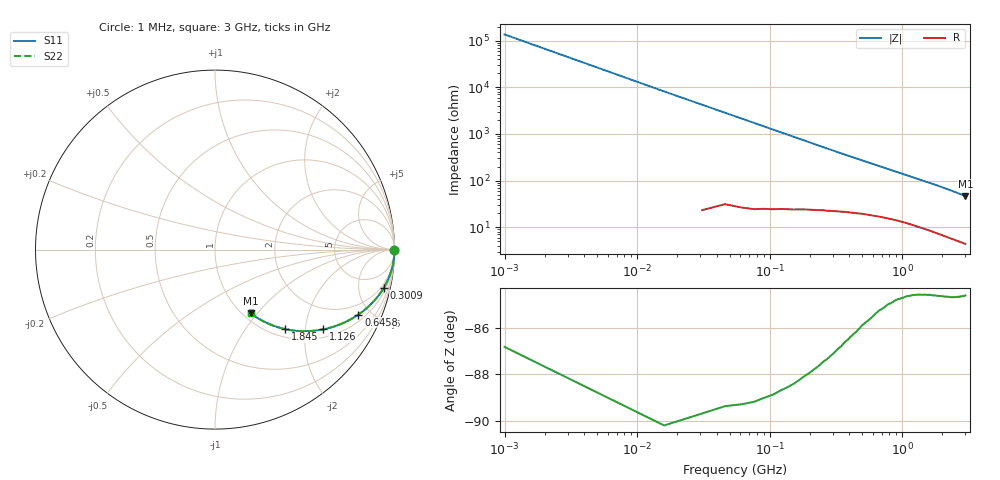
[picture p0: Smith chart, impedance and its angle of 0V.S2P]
!Keysight Technologies,E4991B,MY54301043,A.02.04
!Date: Thu Nov 16 21:16:10 2023
!Data:
!Freq	S11	S21	S12	S22
# Hz S MA R 50
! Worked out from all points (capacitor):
!   201 points, 1 MHz to 3 GHz, reference 50 ohm
!   read as one part in series: C = 1.22 pF near 15.99 MHz
!   lowest |Z| = 46.6 ohm at 3 GHz (marker M1)
!   S11 on the Smith chart (normalised r, x): 1 MHz: open; 300.9 MHz: 1.44, -8.79; 645.8 MHz: 1.35, -4.23; 1.126 GHz: 1.24, -2.51; 1.845 GHz: 1.15, -1.56; 3 GHz: 1.09, -0.93
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1000000  1 -0.0  0.0007395 86.8  0.0007395 86.8  1 -0.0
1.5995e7  1 -0.7  0.01229 89.5  0.01229 89.5  1 -0.7
3.099e7  0.9996 -1.4  0.02374 88.3  0.02374 88.3  0.9996 -1.4
4.5985e7  0.999 -2.0  0.03525 87.3  0.03525 87.3  0.999 -2.0
6.098e7  0.9983 -2.7  0.04665 86.6  0.04665 86.6  0.9983 -2.7
7.5975e7  0.9975 -3.3  0.0581 85.9  0.0581 85.9  0.9975 -3.3
1.05965e8  0.9951 -4.6  0.08074 84.2  0.08074 84.2  0.9951 -4.6
1.35955e8  0.9921 -5.9  0.1031 82.6  0.1031 82.6  0.9921 -5.9
1.65945e8  0.9883 -7.2  0.1251 81.1  0.1251 81.1  0.9883 -7.2
2.1093e8  0.9816 -9.1  0.1574 78.8  0.1574 78.8  0.9816 -9.1
3.009e8  0.9647 -12.6  0.2192 74.5  0.2192 74.5  0.9647 -12.6
3.9087e8  0.9443 -16.0  0.2764 70.5  0.2764 70.5  0.9443 -16.0
5.1083e8  0.9137 -20.1  0.3454 65.7  0.3454 65.7  0.9137 -20.1
6.45785e8  0.8772 -24.4  0.4137 61.0  0.4137 61.0  0.8772 -24.4
8.1073e8  0.8323 -28.9  0.4857 56.0  0.4857 56.0  0.8323 -28.9
1.005665e9  0.7805 -33.7  0.5571 51.0  0.5571 51.0  0.7805 -33.7
1.125625e9  0.7498 -36.3  0.5949 48.3  0.5949 48.3  0.7498 -36.3
1.5005e9  0.6615 -43.4  0.6897 41.2  0.6897 41.2  0.6615 -43.4
1.845385e9  0.5903 -48.6  0.7535 36.0  0.7535 36.0  0.5903 -48.6
2.01033e9  0.5593 -50.8  0.7781 33.8  0.7781 33.8  0.5593 -50.8
2.505165e9  0.477 -56.3  0.8356 28.4  0.8356 28.4  0.477 -56.3
3e9  0.4077 -60.6  0.8755 23.9  0.8755 23.9  0.4077 -60.6
